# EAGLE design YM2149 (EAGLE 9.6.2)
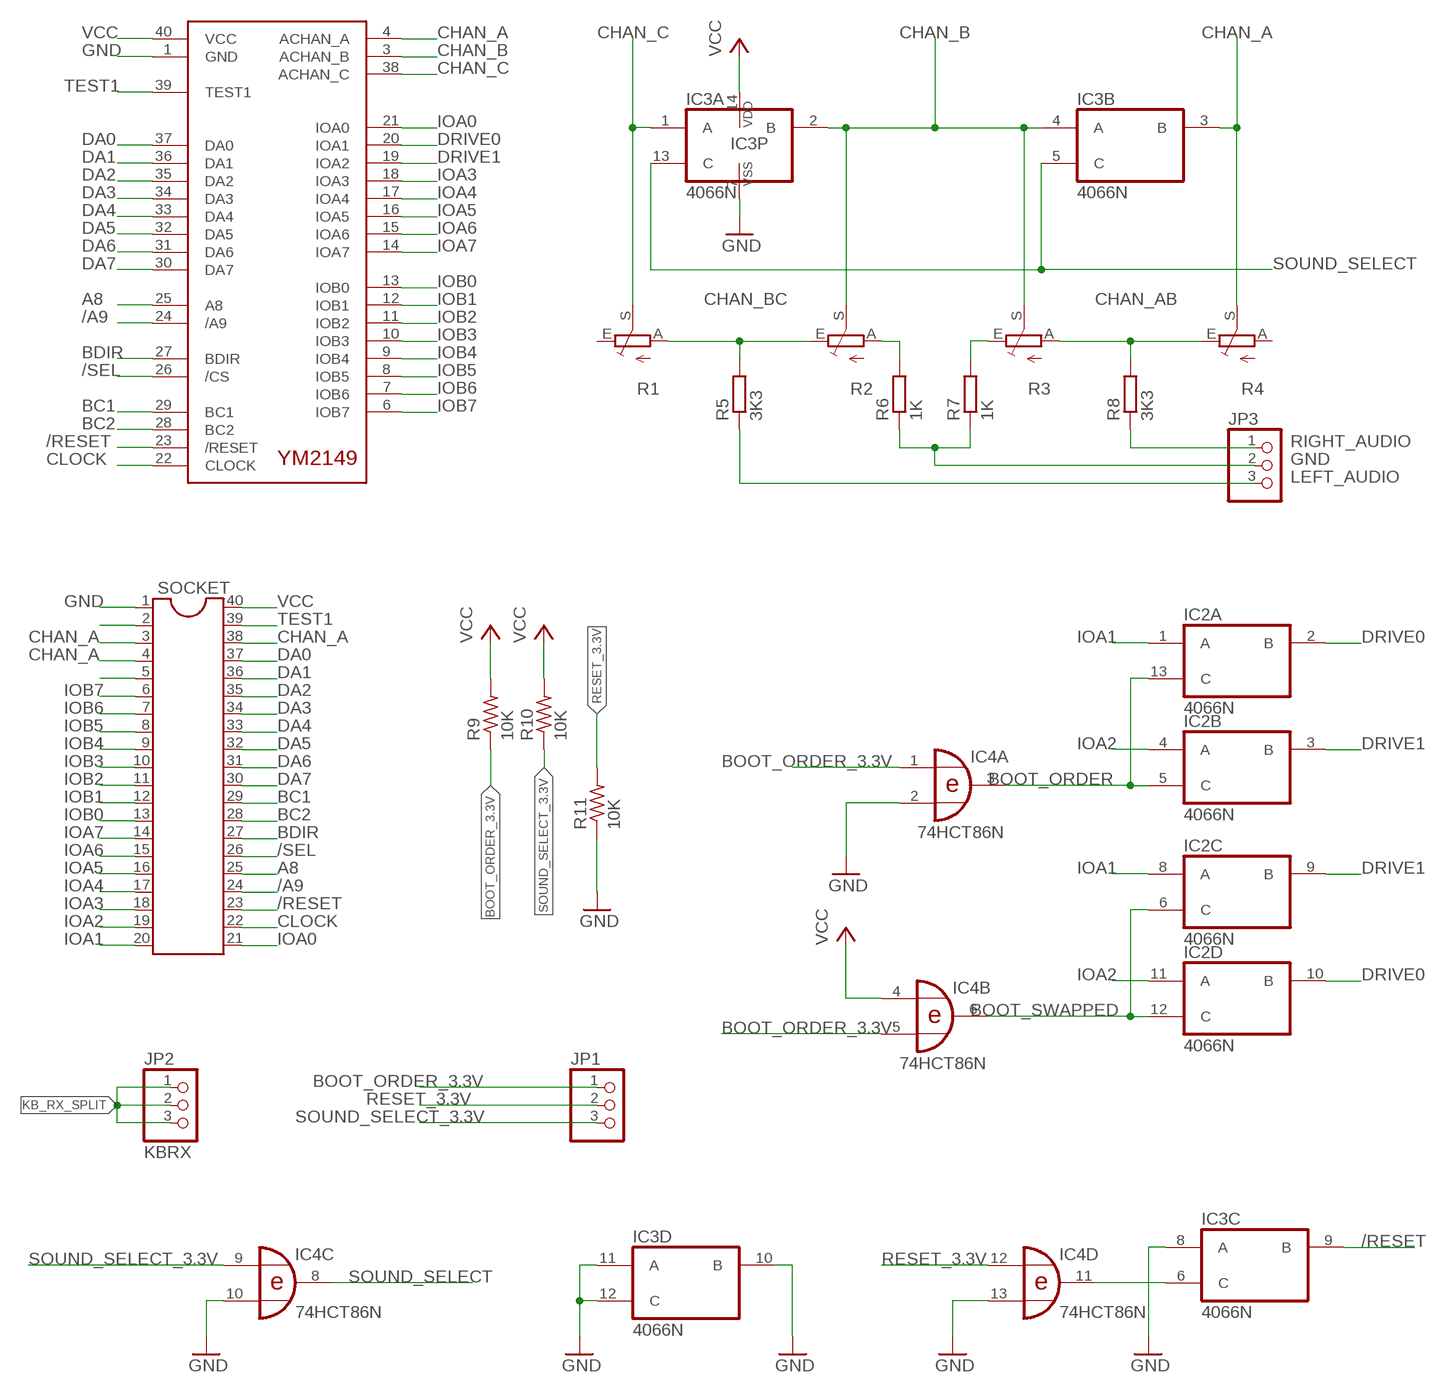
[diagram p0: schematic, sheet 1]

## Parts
IC1  YM2149  [DIL40]
IC2  4066N  [DIL14]
IC3  4066N  [DIL14]
IC4  74HCT86N  [DIL14]
JP1  PINHD-1X3/90  [1X03/90]
JP2  KBRX  PINHD-1X3/90  [1X03/90]
JP3  PINHD-1X3/90  [1X03/90]
R1  TRIM_EU-CA6V  [CA6V]
R2  TRIM_EU-CA6V  [CA6V]
R3  TRIM_EU-CA6V  [CA6V]
R4  TRIM_EU-CA6V  [CA6V]
R5  3K3  R-EU_0204/7  [0204/7]
R6  1K  R-EU_0204/7  [0204/7]
R7  1K  R-EU_0204/7  [0204/7]
R8  3K3  R-EU_0204/7  [0204/7]
R9  10K  R-US_0204/7  [0204/7]
R10  10K  R-US_0204/7  [0204/7]
R11  10K  R-US_0204/7  [0204/7]
SOCKET  DIL40  [DIL40]

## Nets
/A9: IC1.24(/A9) SOCKET.24
/RESET: IC1.23(/RESET) IC3.9(C:B) SOCKET.23
/SEL: IC1.26(/CS) SOCKET.26
A8: IC1.25(A8) SOCKET.25
AB_GND: R3.E R7.2
BC1: IC1.29(BC1) SOCKET.29
BC2: IC1.28(BC2) SOCKET.28
BC_GND: R2.A R6.2
BDIR: IC1.27(BDIR) SOCKET.27
BOOT_ORDER: IC2.5(B:C) IC2.13(A:C) IC4.3(A:O)
BOOT_ORDER_3.3V: IC4.1(A:I0) IC4.5(B:I1) JP1.1 R9.1
BOOT_SWAPPED: IC2.6(C:C) IC2.12(D:C) IC4.6(B:O)
CHAN_A: IC1.4(ACHAN_A) IC3.3(B:B) R4.S SOCKET.3 SOCKET.4 SOCKET.38
CHAN_AB: R3.A R4.E R8.2
CHAN_B: IC1.3(ACHAN_B) IC3.2(A:B) IC3.4(B:A) R2.S R3.S
CHAN_BC: R1.A R2.E R5.2
CHAN_C: IC1.38(ACHAN_C) IC3.1(A:A) R1.S
CLOCK: IC1.22(CLOCK) SOCKET.22
DA0: IC1.37(DA0) SOCKET.37
DA1: IC1.36(DA1) SOCKET.36
DA2: IC1.35(DA2) SOCKET.35
DA3: IC1.34(DA3) SOCKET.34
DA4: IC1.33(DA4) SOCKET.33
DA5: IC1.32(DA5) SOCKET.32
DA6: IC1.31(DA6) SOCKET.31
DA7: IC1.30(DA7) SOCKET.30
DRIVE0: IC1.20(IOA1) IC2.2(A:B) IC2.10(D:B)
DRIVE1: IC1.19(IOA2) IC2.3(B:B) IC2.9(C:B)
GND: IC1.1(GND) IC3.7(P:VSS) IC3.8(C:A) IC3.10(D:B) IC3.11(D:A) IC3.12(D:C) IC4.2(A:I1) IC4.10(C:I1) IC4.13(D:I1) JP3.2 R6.1 R7.1 R11.1 SOCKET.1
IOA0: IC1.21(IOA0) SOCKET.21
IOA1: IC2.1(A:A) IC2.8(C:A) SOCKET.20
IOA2: IC2.4(B:A) IC2.11(D:A) SOCKET.19
IOA3: IC1.18(IOA3) SOCKET.18
IOA4: IC1.17(IOA4) SOCKET.17
IOA5: IC1.16(IOA5) SOCKET.16
IOA6: IC1.15(IOA6) SOCKET.15
IOA7: IC1.14(IOA7) SOCKET.14
IOB0: IC1.13(IOB0) SOCKET.13
IOB1: IC1.12(IOB1) SOCKET.12
IOB2: IC1.11(IOB2) SOCKET.11
IOB3: IC1.10(IOB3) SOCKET.10
IOB4: IC1.9(IOB4) SOCKET.9
IOB5: IC1.8(IOB5) SOCKET.8
IOB6: IC1.7(IOB6) SOCKET.7
IOB7: IC1.6(IOB7) SOCKET.6
KB_RX_SPLIT: JP2.1 JP2.2 JP2.3
LEFT_AUDIO: JP3.3 R5.1
N$2: SOCKET.2
N$5: SOCKET.5
N$7: IC3.6(C:C) IC4.11(D:O)
RESET_3.3V: IC4.12(D:I0) JP1.2 R11.2
RIGHT_AUDIO: JP3.1 R8.1
SOUND_SELECT: IC3.5(B:C) IC3.13(A:C) IC4.8(C:O)
SOUND_SELECT_3.3V: IC4.9(C:I0) JP1.3 R10.1
TEST1: IC1.39(TEST1) SOCKET.39
VCC: IC1.40(VCC) IC3.14(P:VDD) IC4.4(B:I0) R9.2 R10.2 SOCKET.40
Unconnected: R1.E R4.A

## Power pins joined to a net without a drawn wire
GND: IC2.7(P:VSS) IC4.7(P:GND)
VCC: IC2.14(P:VDD) IC4.14(P:VCC)

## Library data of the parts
IC1 = YM2149:YM2149
IC2 IC3 = 40xx:4066: Quad bilateral ANALOG SWITCH
IC4 = 74xx-eu:74*86: Quad 2-input EXCLUSIVE-OR (XOR) gate
JP1-JP3 = pinhead:PINHD-1X3: PIN HEADER
R1-R4 = pot:TRIM_EU-: POTENTIOMETER
R5-R8 = rcl:R-EU_: RESISTOR, European symbol; SPICEPREFIX: R
R9-R11 = rcl:R-US_: RESISTOR, American symbol; SPICEPREFIX: R
SOCKET = ic-package:DIL40: Dual In Line

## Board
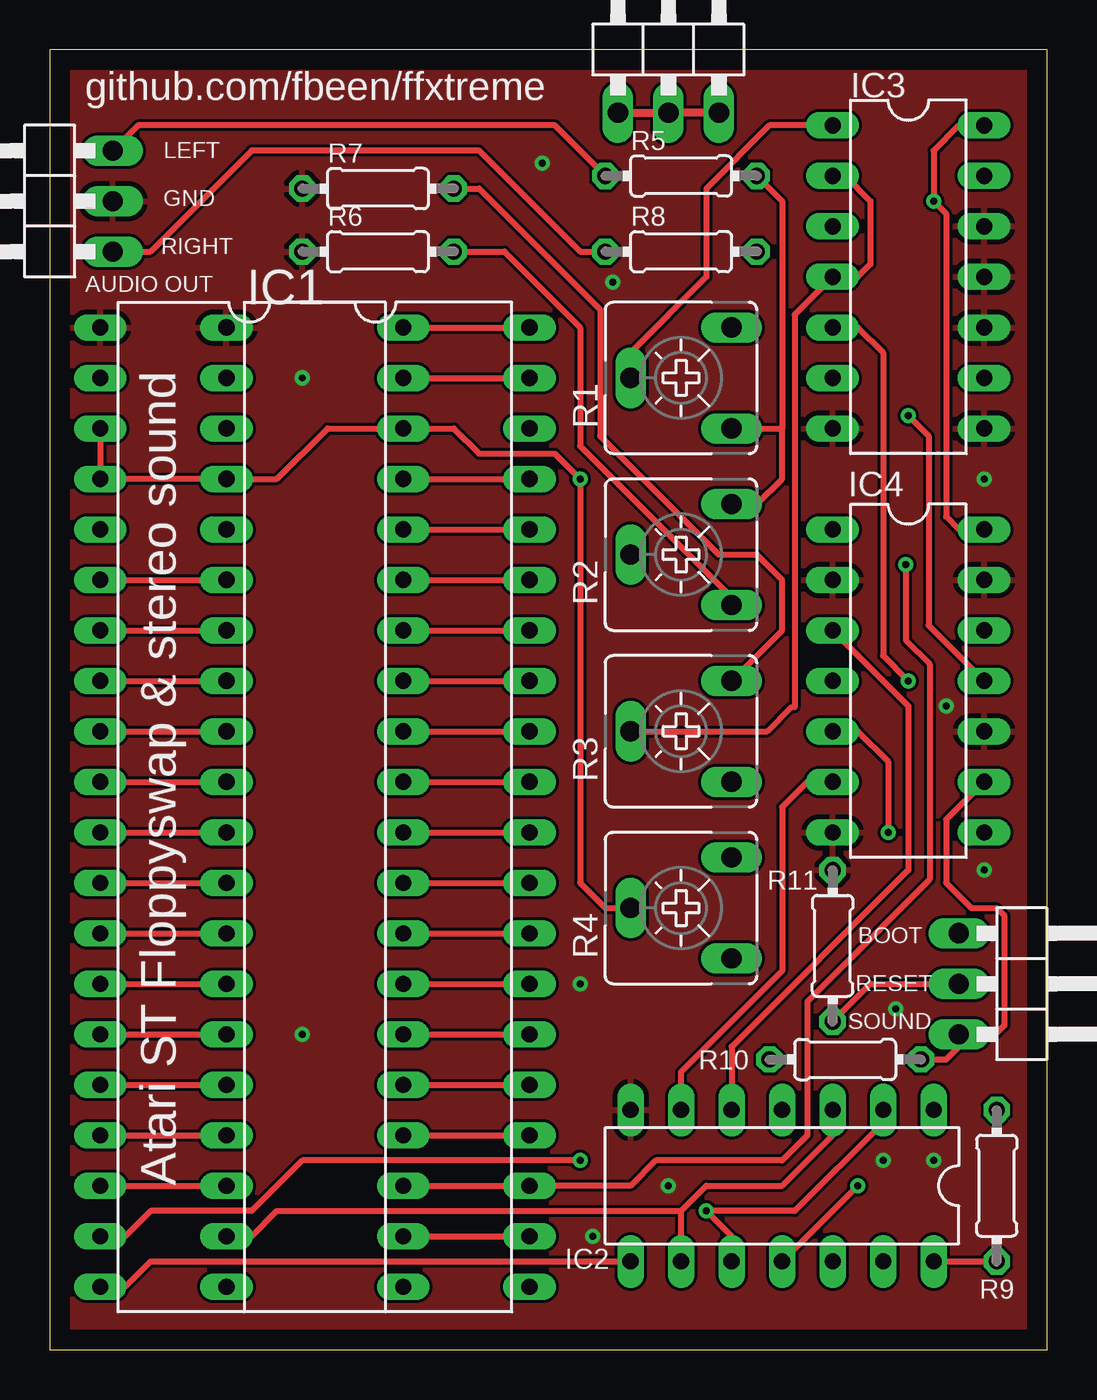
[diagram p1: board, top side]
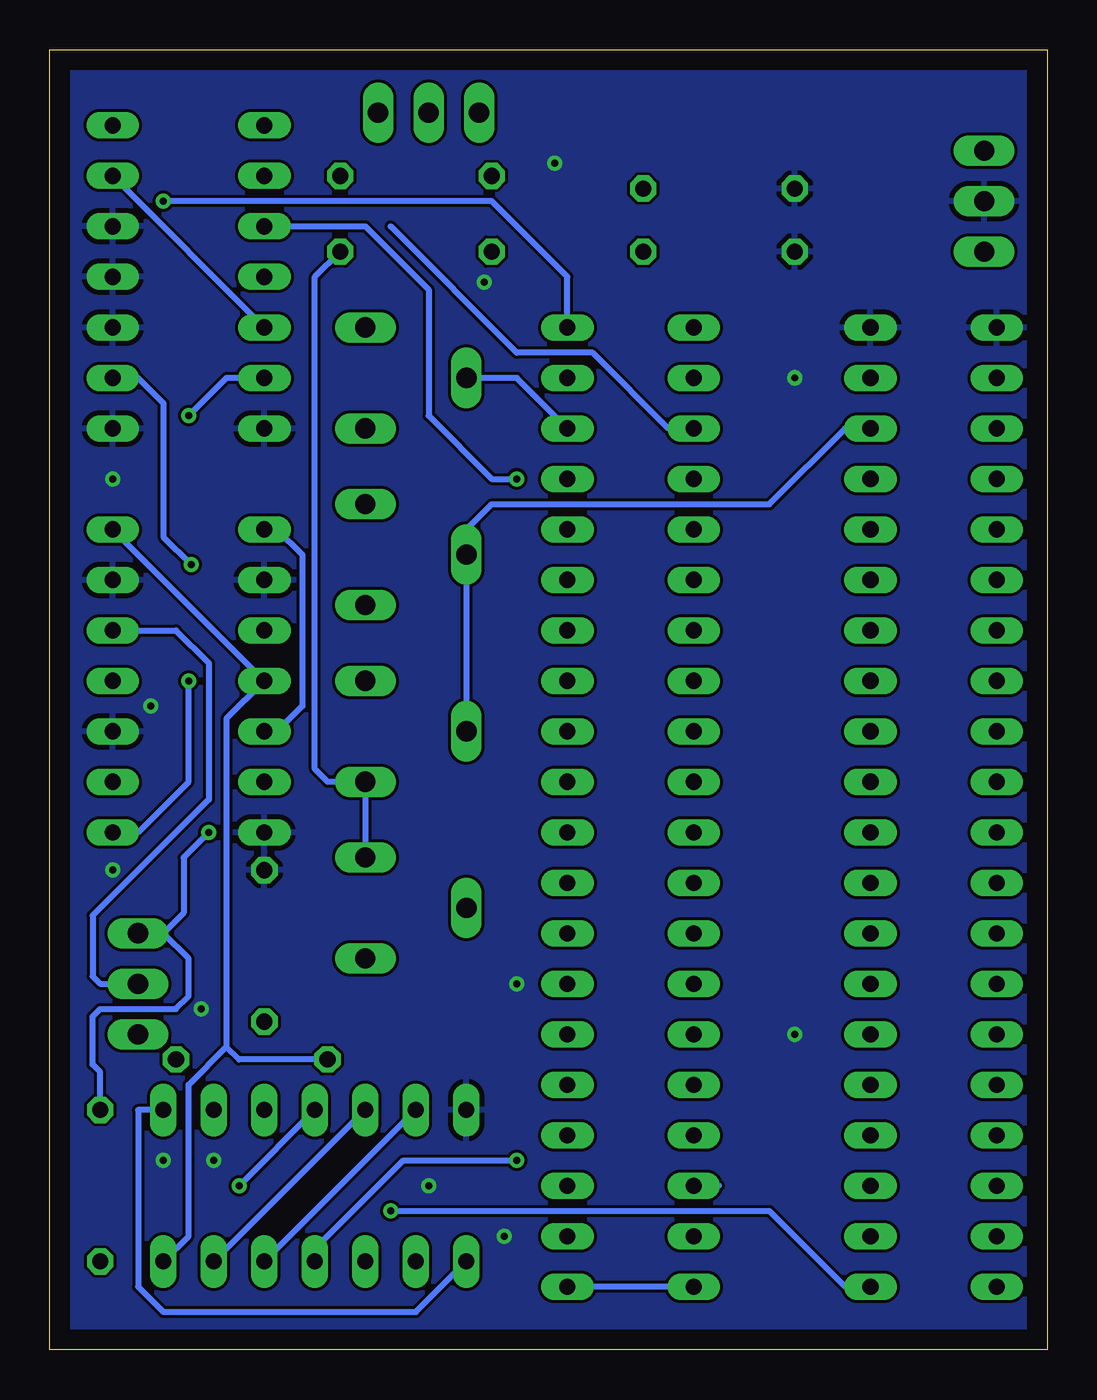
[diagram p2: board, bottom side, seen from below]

Size 50.16 x 65.41 mm. Coordinates in mm from the lower left corner, seen from the top.
Outline: 0,0 50.16,0 50.16,65.41 0,65.4 0,0
Copper layers (1*16): Top 0.035mm / dielectric 1.5mm / Bottom 0.035mm
Design rules "default": minimum track width 6mil, minimum drill 0.35mm, track to track 6mil, track to pad 6mil, pad to pad 6mil, via to via 6mil, smd to smd 6mil, copper to edge 40mil, drill to drill 6mil, minimum pad ring 10mil, minimum via ring 8mil, stop-mask expansion 4mil, vias tented up to drill 0mil, thermal gap 10mil

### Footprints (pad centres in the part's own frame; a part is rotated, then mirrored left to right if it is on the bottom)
DIL40 = drill 0.813 long: 1 -24.13,-7.62; 2 -21.59,-7.62; 3 -19.05,-7.62; 4 -16.51,-7.62; 5 -13.97,-7.62; 6 -11.43,-7.62; 7 -8.89,-7.62; 8 -6.35,-7.62; 9 -3.81,-7.62; 10 -1.27,-7.62; 11 1.27,-7.62; 12 3.81,-7.62; 13 6.35,-7.62; 14 8.89,-7.62; 15 11.43,-7.62; 16 13.97,-7.62; 17 16.51,-7.62; 18 19.05,-7.62; 19 21.59,-7.62; 20 24.13,-7.62; 21 24.13,7.62; 22 21.59,7.62; 23 19.05,7.62; 24 16.51,7.62; 25 13.97,7.62; 26 11.43,7.62; 27 8.89,7.62; 28 6.35,7.62; 29 3.81,7.62; 30 1.27,7.62; 31 -1.27,7.62; 32 -3.81,7.62; 33 -6.35,7.62; 34 -8.89,7.62; 35 -11.43,7.62; 36 -13.97,7.62; 37 -16.51,7.62; 38 -19.05,7.62; 39 -21.59,7.62; 40 -24.13,7.62
DIL14 = drill 0.813 long: 1 -7.62,-3.81; 2 -5.08,-3.81; 3 -2.54,-3.81; 4 0,-3.81; 5 2.54,-3.81; 6 5.08,-3.81; 7 7.62,-3.81; 8 7.62,3.81; 9 5.08,3.81; 10 2.54,3.81; 11 0,3.81; 12 -2.54,3.81; 13 -5.08,3.81; 14 -7.62,3.81
1X03/90 = drill 1.016 long: 1 -2.54,-3.81; 2 0,-3.81; 3 2.54,-3.81
CA6V = drill 1.016 long: A -2.54,-2.54; E 2.54,-2.54; S 0,2.54
0204/7 = drill 0.813 octagon: 1 -3.81,0; 2 3.81,0

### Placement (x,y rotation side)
IC1  16.51,27.3 270 top
IC2  36.83,8.25 180 top
IC3  43.18,53.98 270 top
IC4  43.18,33.66 270 top
JP1  49.53,18.41 270 top
JP2  31.11,66.04 0 top
JP3  -0.64,57.78 90 top
R1  31.75,48.9 90 top
R2  31.75,40.01 90 top
R3  31.75,31.12 90 top
R4  31.75,22.23 90 top
R5  31.75,59.05 0 top
R6  16.51,55.24 0 top
R7  16.51,58.42 0 top
R8  31.75,55.24 0 top
R9  47.62,8.25 270 top
R10  40,14.61 180 top
R11  39.37,20.32 270 top
SOCKET  10.16,27.3 270 top

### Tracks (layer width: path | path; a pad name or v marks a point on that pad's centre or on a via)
/A9
  Top 0.305: SOCKET.24 IC1.24
/RESET  (via drill 0.35)
  Top 0.305: SOCKET.23 IC1.23 29.21,8.25 30.48,9.53 36.83,9.53 38.1,10.79 38.1,17.51 44.25,23.66 44.25,34.49 43.05,35.69 v43.05,39.5
  Bottom 0.305: SOCKET.23 16.51,8.25 | IC3.9 45.72,48.9 44.45,47.62 44.45,40.89 v43.05,39.5
/SEL
  Top 0.305: SOCKET.26 IC1.26
A8
  Top 0.305: SOCKET.25 IC1.25
AB_GND
  Top 0.305: R7.2 21.59,58.42 27.69,52.32 27.69,45.97 33.66,40.01 35.56,40.01 36.83,38.73 36.83,36.2 R3.E
BC1
  Top 0.305: SOCKET.29 IC1.29
BC2
  Top 0.305: SOCKET.28 IC1.28
BC_GND
  Top 0.305: R2.A 34.29,37.85 26.67,45.47 26.67,51.44 22.86,55.24 R6.2
BDIR
  Top 0.305: SOCKET.27 IC1.27
BOOT_ORDER
  Top 0.305: IC2.5 34.29,15.24 43.18,24.13 43.18,32.38 IC4.3
  Bottom 0.305: IC2.5 IC2.13
BOOT_ORDER_3.3V  (via drill 0.35)
  Top 0.305: IC4.5 40.64,31.12 42.16,29.59 v42.16,26.04
  Bottom 0.305: IC4.1 38.73,41.27 37.46,40.01 37.46,32.38 38.73,31.12 IC4.5 | 44.45,20.95 43.43,21.97 43.43,24.77 v42.16,26.04 | JP1.1 44.45,20.95 | R9.1 47.62,13.97 48.01,14.35 48.01,16.76 47.62,17.14 43.81,17.14 43.18,17.78 43.18,19.68 44.45,20.95
BOOT_SWAPPED
  Top 0.305: IC2.6 31.75,13.97 36.83,19.05 36.83,27.3 38.1,28.58 IC4.6
  Bottom 0.305: IC2.6 IC2.12
CHAN_A  (via drill 0.35)
  Top 0.305: SOCKET.3 SOCKET.4 IC1.4 11.43,43.81 13.97,46.35 SOCKET.38 20.32,46.35 21.59,45.09 25.4,45.09 v26.67,43.81 26.67,23.5 27.94,22.23 R4.S
  Bottom 0.305: SOCKET.38 19.05,46.35 22.86,50.16 26.67,50.16 33.02,56.52 | IC3.3 34.29,56.52 31.11,53.34 31.11,46.99 27.94,43.81 v26.67,43.81
CHAN_AB
  Bottom 0.305: R4.E R3.A 36.19,28.58 36.83,29.21 36.83,53.98 R8.2
CHAN_B
  Top 0.305: R3.S 36.08,31.12 37.29,32.33 37.46,32.33 37.46,52.07 IC3.4 40.64,53.98 41.27,54.61 41.27,57.78 40,59.05 IC3.2
  Bottom 0.305: IC1.3 10.16,46.35 13.97,42.55 27.94,42.55 29.21,41.27 R2.S R3.S
CHAN_BC
  Top 0.305: R5.2 36.83,57.78 36.83,46.35 | 36.83,46.35 36.83,43.81 35.56,42.55 R2.E | R1.A 36.83,46.35
CHAN_C
  Top 0.305: R1.S 29.21,50.16 33.02,53.98 33.02,58.42 36.19,61.6 IC3.1
  Bottom 0.305: IC1.38 26.67,48.9 R1.S
CLOCK
  Top 0.305: SOCKET.22 IC1.22
DA0
  Top 0.305: SOCKET.37 IC1.37
DA1
  Top 0.305: SOCKET.36 IC1.36
DA2
  Top 0.305: SOCKET.35 IC1.35
DA3
  Top 0.305: SOCKET.34 IC1.34
DA4
  Top 0.305: SOCKET.33 IC1.33
DA5
  Top 0.305: SOCKET.32 IC1.32
DA6
  Top 0.305: SOCKET.31 IC1.31
DA7
  Top 0.305: SOCKET.30 IC1.30
DRIVE0  (via drill 0.35)
  Top 0.305: IC2.2 41.91,11.43 37.46,6.98 v33.02,6.98 34.29,5.71 IC2.10
  Bottom 0.305: IC1.20 10.16,3.17 13.97,6.98 v33.02,6.98
DRIVE1
  Top 0.305: IC1.19 10.16,5.71 11.43,6.98 31.75,6.98 | IC2.9 31.75,6.98 | IC2.3 39.37,10.79 36.83,8.25 33.02,8.25 31.75,6.98
GND  (via drill 0.35)
  other vias: 12.7,48.9 12.7,15.88 26.67,18.41 46.99,43.81 24.76,59.69 27.3,5.71 45.08,32.38 46.99,24.13 42.55,17.14 41.91,9.53 44.45,9.53 28.32,53.72 31.11,8.25
  pour Top: 0,65.41 50.16,65.41 50.16,0.13 0,0.13
  pour Bottom: 0,65.41 50.16,65.41 50.16,0 0,0
IOA0
  Bottom 0.305: SOCKET.21 IC1.21
IOA1
  Top 0.305: SOCKET.20 3.81,3.17 5.08,4.45 IC2.8
  Bottom 0.305: IC2.1 45.72,12.07 45.72,3.17 44.45,1.9 31.75,1.9 IC2.8
IOA2  (via drill 0.35)
  Top 0.305: v26.67,9.53 12.7,9.53 10.16,6.98 5.08,6.98 3.81,5.71 SOCKET.19 | v40.64,8.25 IC2.11
  Bottom 0.305: IC2.11 36.83,5.08 32.39,9.53 v26.67,9.53 | IC2.4 v40.64,8.25
IOA3
  Top 0.305: SOCKET.18 IC1.18
IOA4
  Top 0.305: SOCKET.17 IC1.17
IOA5
  Top 0.305: SOCKET.16 IC1.16
IOA6
  Top 0.305: SOCKET.15 IC1.15
IOA7
  Top 0.305: SOCKET.14 IC1.14
IOB0
  Top 0.305: SOCKET.13 IC1.13
IOB1
  Top 0.305: SOCKET.12 IC1.12
IOB2
  Top 0.305: SOCKET.11 IC1.11
IOB3
  Top 0.305: SOCKET.10 IC1.10
IOB4
  Top 0.305: SOCKET.9 IC1.9
IOB5
  Top 0.305: SOCKET.8 IC1.8
IOB6
  Top 0.305: SOCKET.7 IC1.7
IOB7
  Top 0.305: SOCKET.6 IC1.6
KB_RX_SPLIT
  Top 0.406: JP2.1 JP2.2 JP2.3
LEFT_AUDIO
  Top 0.305: R5.1 25.4,61.6 4.44,61.6 JP3.3
N$7  (via drill 0.35)
  Top 0.305: IC4.11 44.2,36.45 44.2,45.97 v43.18,46.99
  Bottom 0.305: IC3.6 41.27,48.9 v43.18,46.99
RESET_3.3V
  Top 0.305: R11.2 41.27,18.41 JP1.2
  Bottom 0.305: JP1.2 47.62,18.41 48.01,18.8 48.01,21.84 42.16,27.69 42.16,34.54 43.81,36.2 IC4.12
RIGHT_AUDIO
  Top 0.305: R8.1 26.67,55.24 21.59,60.32 10.16,60.32 5.08,55.24 JP3.1
SOUND_SELECT  (via drill 0.35)
  Top 0.305: IC3.5 40.64,51.44 41.91,50.16 41.91,34.92 v43.18,33.66
  Bottom 0.305: IC4.8 45.72,26.04 43.18,28.58 v43.18,33.66 | IC3.13 IC3.5
SOUND_SELECT_3.3V
  Top 0.305: IC4.9 45.08,26.67 45.08,23.5 46.35,22.23 47.62,22.23 48.01,21.84 48.01,16.32 47.56,15.88 JP1.3 45.72,15.24 45.08,14.61 R10.1
TEST1
  Top 0.305: SOCKET.39 IC1.39
VCC  (via drill 0.35)
  Top 0.305: SOCKET.40 IC1.40 | IC4.14 45.72,41.27 45.08,41.91 45.08,57.15 v44.45,57.78 44.45,60.32 45.72,61.6 IC3.14 | IC2.14 R9.2
  Bottom 0.305: IC1.40 24.13,53.98 27.94,57.78 v44.45,57.78 | 41.27,15.24 43.18,13.34 43.18,5.71 IC2.14 | IC4.14 IC4.4 41.27,31.75 41.27,15.24 | 41.27,15.24 40.64,14.61 R10.2

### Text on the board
tNames: github.com/fbeen/ffxtreme | LEFT | GND | RIGHT | AUDIO OUT | BOOT | RESET | SOUND | Atari ST Floppyswap & stereo sound
tValues: SPLIT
